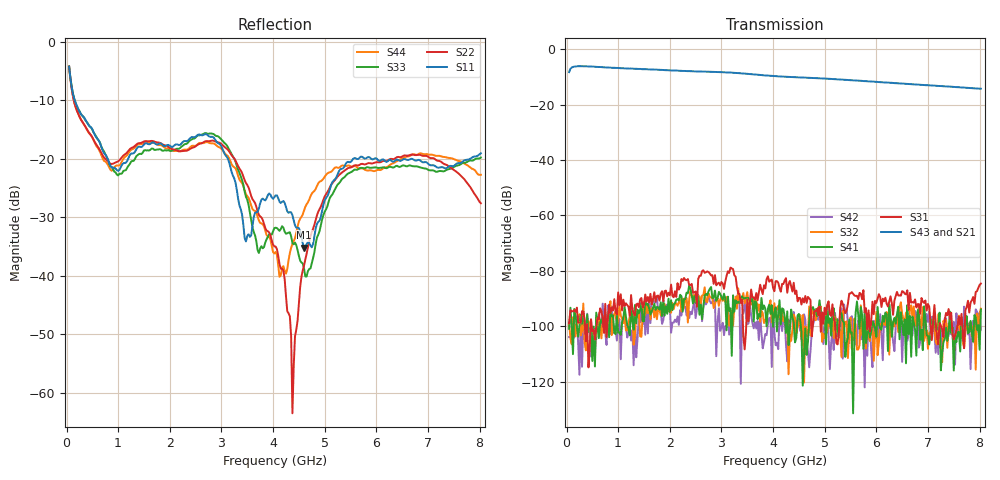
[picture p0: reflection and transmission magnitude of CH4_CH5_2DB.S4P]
!Agilent Technologies,E5071C,MY46316741,A.11.02
!Date: Mon Jun 01 11:48:05 2026
!Data & Calibration Information:
!1:CH4 INPUT 2:CH4 OUTPUT 3:CH5 INPUT 4:CH5 OUTPUT
!Freq	S11:SOLT4(ON)	S12:SOLT4(ON)	S13:SOLT4(ON)	S14:SOLT4(ON)
!	S21:SOLT4(ON)	S22:SOLT4(ON)	S23:SOLT4(ON)	S24:SOLT4(ON)
!	S31:SOLT4(ON)	S32:SOLT4(ON)	S33:SOLT4(ON)	S34:SOLT4(ON)
!	S41:SOLT4(ON)	S42:SOLT4(ON)	S43:SOLT4(ON)	S44:SOLT4(ON)
!PortZ  Port1:50+j0  Port2:50+j0  Port3:50+j0  Port4:50+j0
!Above PortZ is port z conversion or system Z0 setting when saving the data.
!When reading, reference impedance value at option line is always used.
# Hz S dB R 50
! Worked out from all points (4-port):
!   320 points, 50 MHz to 8.025 GHz, reference 50 ohm
!   strongest paths, dB at 50 MHz, 2.05 GHz, 4.05 GHz, 6.05 GHz, 8.025 GHz:
!     S43: -8.2, -7.6, -9.7, -11.8, -14.2
!     S21: -8.3, -7.8, -9.9, -12.1, -14.4
!     S31: -99.0, -89.0, -83.7, -88.4, -84.6
!     S41: -100.9, -94.2, -93.2, -99.2, -93.9
!     S32: -98.7, -91.6, -96.7, -105.8, -93.7
!     S42: -103.9, -98.7, -106.8, -104.3, -101.2
!   lowest |S11| = -35.2 dB at 4.6 GHz (marker M1), VSWR 1.04, Z = 51.4 + j1.07 ohm
!   |S11| at or under -10 dB: 158.4 MHz to end of sweep
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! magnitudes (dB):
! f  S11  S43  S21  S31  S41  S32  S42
! 50 MHz  -4.2  -8.2  -8.3  -99.0  -100.9  -98.7  -103.9
! 3.25 GHz  -23.4  -8.5  -8.7  -81.6  -94.8  -92.9  -93.1
! 4.2 GHz  -27.2  -9.9  -10.1  -84.7  -93.8  -98.3  -97.5
! 4.375 GHz  -29.6  -10.0  -10.3  -87.5  -96.7  -101.2  -96.8
! 4.6 GHz  -35.2  -10.2  -10.4  -91.4  -110.2  -120.3  -95.7
! 5.575 GHz  -19.8  -11.2  -11.4  -88.9  -103.8  -97.3  -100.5
! 8.025 GHz  -19.1  -14.2  -14.4  -84.6  -93.9  -93.7  -101.2
